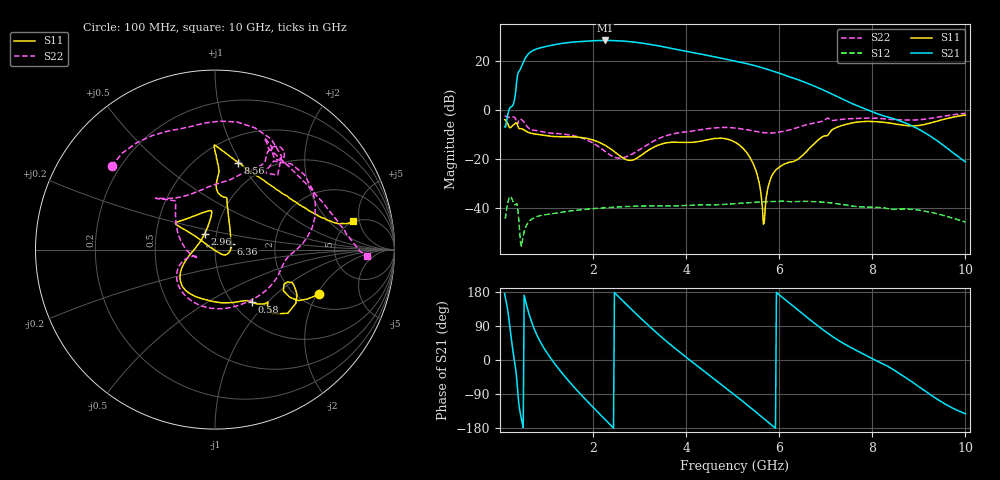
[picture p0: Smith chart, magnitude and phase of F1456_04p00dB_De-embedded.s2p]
! Integrated Device Technology
! Corporate Headquarters
! 6024 Silver Creek Valley Road
! San Jose, CA 95138  USA
! Phone:  1-408-284-8200
! Toll Free:  1-800-223-1366
! Webpage:  http://www.idt.com/
! Timing and RF Division
! 515 Groton Road, Suite 102
! Westford, MA 01886-6024
! Device:  F1456
! Description: 6-bit 0.5 dB Transmit Variable Gain Amplifier
! Frequency:  2100.0 -  2950.00 MHz
! Package:  6x6 mm Thin QFN Plastic Package: 28 pin
! State:  8
! Atten State:  4.0 dB
! Voltage:  +5.00 Volts
! Current:  215.492 mA
! Data:  The device was measured on a the F1455 evaluation board which has
!  individual transmission lines to the RF pins.  Data was collected
!  using a calibrated network analyzer.  The evaluation board was
!  de-embedded using a TRL calibration technique.
!  The reference plane is the edge of the package pin.
!  Pin  1 = CSb
!  Pin  2 = DATA
!  Pin  3 = CLK
!  Pin  4 = RSET
!  Pin  5 = GND
!  Pin  6 = RFIN  = Port 1
!  Pin  7 = GND
!  Pin  8 = NC
!  Pin  9 = NC
!  Pin 10 = NC
!  Pin 11 = NC
!  Pin 12 = NC
!  Pin 13 = NC
!  Pin 14 = /STBY
!  Pin 15 = GND
!  Pin 16 = RFOUT  = Port 2
!  Pin 17 = GND
!  Pin 18 = NC
!  Pin 19 = NC
!  Pin 20 = NC
!  Pin 21 = GND
!  Pin 22 = NC
!  Pin 23 = GND
!  Pin 24 = NC
!  Pin 25 = NC
!  Pin 26 = NC
!  Pin 27 = GND
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# GHz S dB R 50
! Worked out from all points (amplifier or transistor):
!   496 points, 100 MHz to 10 GHz, reference 50 ohm
!   highest |S21| = 28.3 dB at 2.26 GHz (marker M1)
!   |S21| within 3 dB of that: 869.2 MHz to 3.623 GHz (2.754 GHz wide, 123 % of centre)
!   unconditionally stable (mu >= 1): start of sweep to end of sweep
!   at 1.74 GHz: K = 2.06, MAG = 28.4 dB, |S12| = -40.7 dB
!   at 5.06 GHz: K = 3.38, MAG = 20.8 dB, |S12| = -38.2 dB
!   at 10 GHz: K = 121.56, MAG = -11.6 dB, |S12| = -45.7 dB
!   S11 on the Smith chart (normalised r, x): 100 MHz: 2.56, -2.09; 580 MHz: 1.22, -0.82; 2.96 GHz: 0.88, +0.16; 6.36 GHz: 1.19, +0.07; 8.56 GHz: 0.75, +0.98; 10 GHz: 4.92, +4.02
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0.1  -3.99 -22.8  -6.88 175.5  -43.86 43.0  -2.61 141.1
0.34  -5.34 -33.6  7.90 -26.1  -38.54 -142.7  -3.89 54.5
0.42  -7.62 -44.6  15.98 -128.2  -48.78 134.8  -3.89 48.2
0.58  -8.90 -54.8  22.09 140.9  -46.69 -178.7  -6.71 0.9
0.78  -9.94 -65.6  24.76 69.7  -43.57 125.3  -8.43 -23.4
0.96  -10.44 -80.0  25.70 28.6  -42.77 92.3  -9.14 -51.7
1.14  -10.84 -94.9  26.45 -3.9  -42.30 70.7  -9.55 -77.5
1.48  -10.97 -117.4  27.44 -55.9  -41.28 41.4  -10.19 -119.2
1.76  -11.30 -132.5  27.90 -93.9  -40.67 22.1  -11.47 -142.9
2.26  -14.49 -156.2  28.27 -157.2  -39.85 -7.3  -16.96 -163.8
2.58  -18.78 179.1  28.10 163.3  -39.50 -24.7  -19.69 -155.4
2.96  -19.51 122.0  27.43 117.8  -39.24 -44.5  -16.66 -173.7
3.4  -14.42 96.3  26.09 68.1  -39.14 -66.0  -11.83 147.2
4.04  -13.27 111.7  23.69 3.5  -38.89 -93.0  -8.93 130.2
4.54  -11.86 142.0  21.87 -44.3  -38.73 -114.7  -7.51 137.8
5.06  -13.26 147.0  19.86 -93.8  -38.22 -136.5  -7.43 137.8
5.64  -40.01 171.2  17.12 -151.8  -37.50 -166.9  -9.25 120.5
6.36  -20.55 19.2  12.58 136.4  -37.37 150.3  -7.39 73.2
6.7  -14.77 64.9  10.10 102.5  -37.34 128.1  -5.57 61.9
8.36  -5.36 83.4  -3.05 -18.5  -40.40 52.3  -3.85 62.6
8.56  -5.99 75.0  -4.26 -33.9  -40.47 47.8  -4.03 57.6
10  -2.10 11.5  -21.19 -142.0  -45.68 -28.8  -1.46 -2.5
